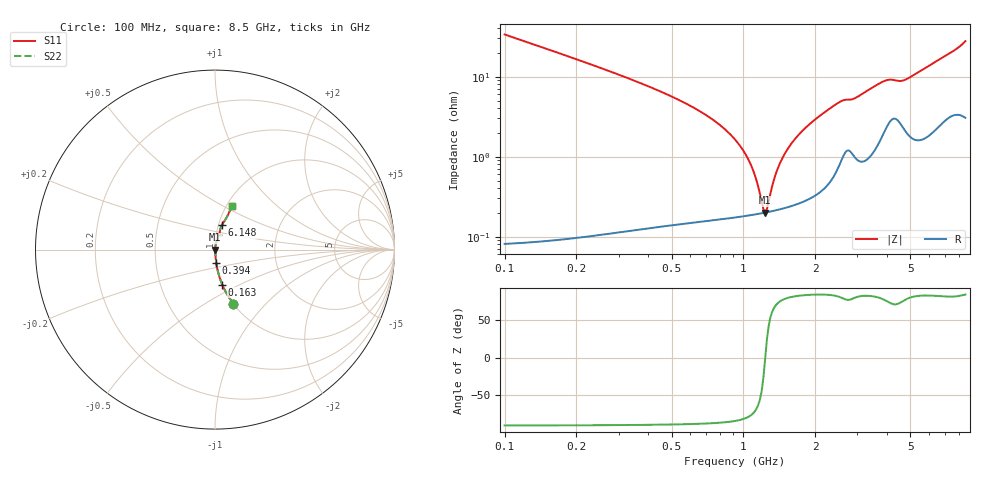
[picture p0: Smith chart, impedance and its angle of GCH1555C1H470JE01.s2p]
!Murata Part Number: GCH1555C1H470JE01
!These Parameters are Measured in Series Mode Connection
!Data Generated on Jun 19, 2026
!  o--ll--o
!Port1  Port2
!  o------o
!Operation Temp=25[degC], DC Bias Voltage=0[V]
!Freq. Start=100[MHz] Stop=9[GHz] 401[Steps]
# Hz S RI R 50
!Freq.(Hz) S11(Real) S11(Imag) S21(Real) S21(Imag) S12(Real) S12(Imag) S22(Real) S22(Imag)
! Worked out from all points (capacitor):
!   401 points, 100 MHz to 8.5 GHz, reference 50 ohm
!   read as one part in series: C = 47.1 pF near 142 MHz
!   lowest |Z| = 200 mohm at 1.234 GHz (marker M1)
!   series resonance near 1.234 GHz, so ESL is about 350 pH
!   S11 on the Smith chart (normalised r, x): 100 MHz: 1.00, -0.67; 163 MHz: 1.00, -0.41; 394 MHz: 1.00, -0.15; 6.148 GHz: 1.04, +0.29; 8.5 GHz: 1.06, +0.55
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1e8  0.1022 -0.3016  0.8978 0.3016  0.8978 0.3016  0.1022 -0.3016
1.63e8  0.0407 -0.1954  0.9593 0.1954  0.9593 0.1954  0.0407 -0.1954
2.68e8  0.0153 -0.1182  0.9847 0.1182  0.9847 0.1182  0.0153 -0.1182
3.94e8  0.00713 -0.0763  0.9929 0.0763  0.9929 0.0763  0.00713 -0.0763
9.61e8  0.00195 -0.0139  0.998 0.0139  0.998 0.0139  0.00195 -0.0139
1.066e9  0.00191 -0.00809  0.9981 0.00809  0.9981 0.00809  0.00191 -0.00809
1.192e9  0.00196 -0.00191  0.998 0.00191  0.998 0.00191  0.00196 -0.00191
1.234e9  0.00199 -1.4e-06  0.998 1.4e-06  0.998 1.4e-06  0.00199 -1.4e-06
1.276e9  0.00204 0.00185  0.998 -0.00185  0.998 -0.00185  0.00204 0.00185
1.381e9  0.00218 0.00627  0.9978 -0.00627  0.9978 -0.00627  0.00218 0.00627
1.507e9  0.00242 0.0112  0.9976 -0.0112  0.9976 -0.0112  0.00242 0.0112
1.738e9  0.00303 0.0197  0.997 -0.0197  0.997 -0.0197  0.00303 0.0197
2.095e9  0.00462 0.0321  0.9954 -0.0321  0.9954 -0.0321  0.00462 0.0321
2.536e9  0.0103 0.0468  0.9897 -0.0468  0.9897 -0.0468  0.0103 0.0468
2.914e9  0.0125 0.0512  0.9875 -0.0512  0.9875 -0.0512  0.0125 0.0512
3.796e9  0.0237 0.08  0.9763 -0.08  0.9763 -0.08  0.0237 0.08
4.3e9  0.0356 0.0796  0.9644 -0.0796  0.9644 -0.0796  0.0356 0.0796
4.699e9  0.0287 0.083  0.9713 -0.083  0.9713 -0.083  0.0287 0.083
5.707e9  0.031 0.119  0.969 -0.119  0.969 -0.119  0.031 0.119
6.148e9  0.0381 0.1349  0.9619 -0.1349  0.9619 -0.1349  0.0381 0.1349
7.114e9  0.0587 0.1687  0.9413 -0.1687  0.9413 -0.1687  0.0587 0.1687
8.5e9  0.0944 0.2423  0.9056 -0.2423  0.9056 -0.2423  0.0944 0.2423
